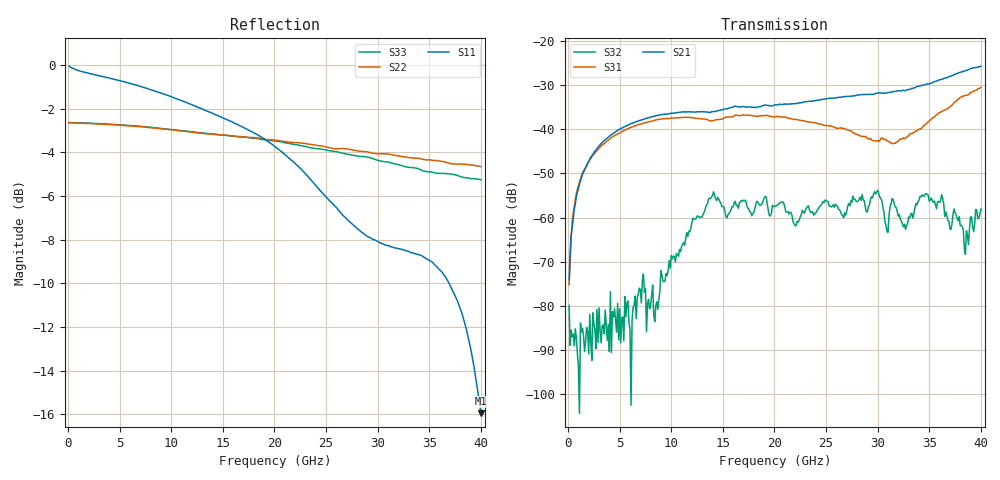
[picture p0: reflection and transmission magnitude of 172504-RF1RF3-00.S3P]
!  3-Port S-parameters saved by WinCal
! VAR MeasName=S-Parameters (CALIBRATED_DATA) read from VNA (N5245A)
! VAR MeasDate=2017-3-15 11:05:20
! VAR NAME=172504-RF1RF3-00
! VAR FILENAME=172504-RF1RF3-00.S3P
! VAR DATE=2017-3-15 11:05:20
! VAR PHYS_PORTS=1,2,3
# Hz S DB R 50
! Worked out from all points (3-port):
!   400 points, 100 MHz to 40 GHz, reference 50 ohm
!   strongest paths, dB at 100 MHz, 10.1 GHz, 20.1 GHz, 30.1 GHz, 40 GHz:
!     S21: -74.0, -36.3, -34.4, -31.7, -25.7
!     S31: -75.2, -37.5, -37.1, -42.7, -30.5
!     S32: -79.9, -69.3, -57.3, -54.5, -58.0
!   lowest |S11| = -15.9 dB at 40 GHz (marker M1), VSWR 1.38, Z = 37.8 - j6.91 ohm
!   |S11| at or under -10 dB: 36.92 GHz to end of sweep
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1e8  -0.06 -1.8  -77.81 56.7  -75.32 134.9
     -74.05 98.1  -2.66 179.8  -84.59 85.7
     -75.25 93.7  -79.93 -79.3  -2.64 179.8
8e8  -0.23 -12.1  -55.35 93.6  -54.58 88.2
     -55.32 93.3  -2.66 178.3  -90.85 -54.3
     -54.52 88.2  -87.14 131.6  -2.65 178.3
3.3e9  -0.53 -45.7  -43.03 67.0  -43.65 55.4
       -42.98 67.1  -2.72 173.0  -83.20 115.4
       -43.63 55.6  -84.52 96.8  -2.70 173.2
8.7e9  -1.24 -107.3  -36.84 30.4  -37.77 9.8
       -36.80 30.5  -2.91 161.9  -79.68 -172.0
       -37.77 9.3  -80.76 151.0  -2.89 162.4
1.18e10  -1.79 -136.1  -36.02 14.2  -37.29 -14.7
         -36.02 14.3  -3.07 155.7  -63.56 172.5
         -37.30 -14.8  -63.15 171.8  -3.05 156.3
2.01e10  -3.76 149.9  -34.48 -9.9  -37.10 -61.2
         -34.41 -9.0  -3.45 137.9  -56.79 73.4
         -37.15 -60.8  -57.27 71.5  -3.48 138.5
2.96e10  -8.00 15.5  -31.85 -42.0  -42.30 -99.9
         -32.03 -41.3  -4.05 114.1  -54.23 61.8
         -42.55 -100.0  -54.61 64.0  -4.31 113.9
3.62e10  -9.47 -80.7  -28.31 -67.3  -35.56 -85.6
         -28.63 -65.4  -4.41 94.9  -56.09 32.3
         -35.98 -83.3  -54.80 34.0  -4.97 95.0
3.85e10  -11.93 -115.4  -26.38 -83.0  -32.06 -102.7
         -26.72 -80.2  -4.55 87.8  -65.44 94.5
         -32.31 -100.1  -68.31 93.7  -5.17 87.3
4e10  -15.95 -146.0  -25.39 -96.4  -30.33 -117.3
      -25.67 -93.4  -4.66 82.6  -58.51 124.4
      -30.48 -112.5  -58.03 126.0  -5.26 82.6
